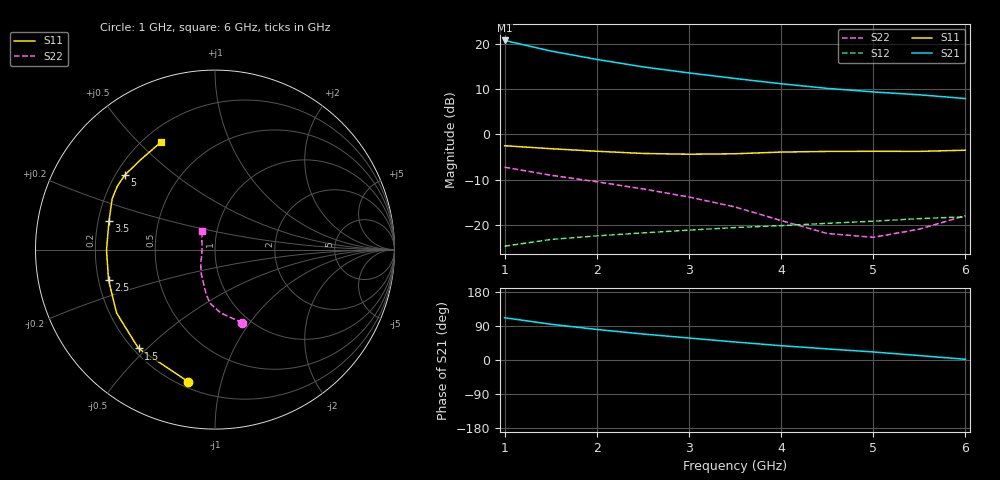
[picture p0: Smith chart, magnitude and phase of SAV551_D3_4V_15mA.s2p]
! Created Mon Oct 27 14:31:09 2008
# hz S ma R 50
! 2 Port Network Data from SP1.SP block
! freq  magS11  angS11  magS21  angS21  magS12  angS12  magS22  angS22
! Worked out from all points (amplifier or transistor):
!   11 points, 1 GHz to 6 GHz, reference 50 ohm
!   highest |S21| = 20.8 dB at 1 GHz (marker M1)
!   |S21| within 3 dB of that: start of sweep to 1.68 GHz
!   unconditionally stable (mu >= 1): 4.65 GHz to end of sweep
!   at 1.5 GHz: K = 0.45, MSG = 20.9 dB, |S12| = -23.2 dB
!   at 3.5 GHz: K = 0.89, MSG = 16.5 dB, |S12| = -20.6 dB
!   at 6 GHz: K = 1.08, MAG = 11.4 dB, |S12| = -18.2 dB
!   S11 on the Smith chart (normalised r, x): 1 GHz: 0.23, -0.79; 1.5 GHz: 0.22, -0.47; 2.5 GHz: 0.24, -0.13; 3.5 GHz: 0.24, +0.12; 5 GHz: 0.24, +0.34; 6 GHz: 0.27, +0.58
1e9  0.751 -101.5  10.97 111.5  0.0581 39.4  0.4344 -69.6
1.5e9  0.6961 -127.8  8.386 94.4  0.06889 31.1  0.3543 -85.0
2e9  0.6523 -147.2  6.771 80.6  0.07552 25.0  0.2997 -95.4
2.5e9  0.6168 -164.0  5.598 68.6  0.08148 20.7  0.25 -101.6
3e9  0.6044 -179.7  4.798 58.0  0.08743 17.8  0.2033 -108.0
3.5e9  0.6118 164.9  4.164 47.5  0.09331 13.9  0.1577 -118.8
4e9  0.6389 153.8  3.641 37.8  0.098 10.6  0.1116 -135.9
4.5e9  0.6492 146.8  3.236 29.3  0.104 7.8  0.08028 -156.9
5e9  0.6517 140.1  2.957 21.3  0.1098 4.4  0.07281 174.3
5.5e9  0.6502 129.0  2.748 11.7  0.1172 0.9  0.08956 144.8
6e9  0.6695 117.0  2.498 1.9  0.1229 -3.7  0.1263 124.8
